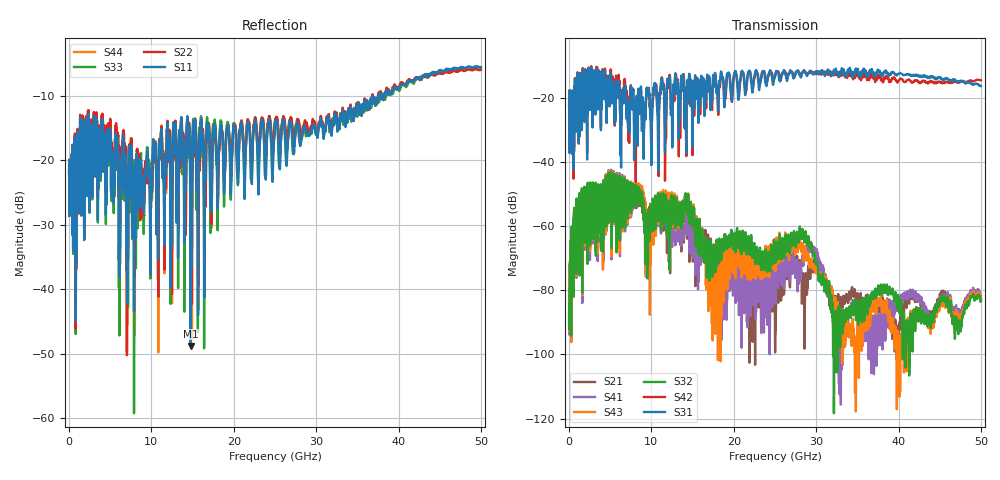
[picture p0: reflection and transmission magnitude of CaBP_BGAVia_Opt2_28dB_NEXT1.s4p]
!* Samtec Inc. NovaRay Examax Flyover System  *
!*  REV DATE  = 08/08/18  *
!*  TYPE  = TOUCHSTONE  *
!*  PORTS  = 4 port  *
!*  UNITS  = GHz  *
!*  DATA RANGE = DC  to 50 GHz; 10 MHz Step  *
!*  PARAMETER  = S  *
!*  FORMAT  = Real-Imaginary  *
!*  REFERENCE  = 50 ohms  *
!*  SOURCE  = HFSS  *
!*  VALIDATED  = No  *
!*  MANUFACTURER = SAMTEC  *
!*  INTERCONNECT = NVAx to EBCx to EBCx to NVAx  *
!*  [Full Channel NVAx to EBCx to EBCx to NVAx  with PCB Trace and BGA Via]  *
!*  BOUNDARY A  = Silicon BGA Ball Pad  *
!*  BOUNDARY B  = Silicon BGA Ball Pad  *
!*  NVAx (end a) ->>- (end b) NVAx  *
!*  Port 01 ->>- Port 02  *
!*  Port 03 ->>- Port 04  *
!***************************** CHANNEL MODEL ******************************************
# GHz S RI R 50
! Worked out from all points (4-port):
!   5000 points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, 10 MHz to 50 GHz, reference 50 ohm
!   strongest paths, dB at 10 MHz, 12.51 GHz, 25.01 GHz, 37.51 GHz, 50 GHz:
!     S31: -23.1, -28.5, -13.0, -11.3, -16.4
!     S42: -23.1, -22.9, -13.4, -12.9, -14.5
!     S32: -87.8, -59.5, -69.8, -78.9, -83.4
!     S43: -88.9, -57.6, -71.3, -83.6, -82.5
!     S41: -90.3, -63.2, -82.9, -89.0, -81.8
!     S21: -88.4, -62.3, -96.7, -84.9, -82.9
!   lowest |S11| = -48.8 dB at 14.75 GHz (marker M1), VSWR 1.01, Z = 49.7 - j0.221 ohm
!   |S11| at or under -10 dB: start of sweep to 37.51 GHz; 37.83997 GHz to 38.00552 GHz (165.6 MHz wide, 0.437 % of centre); 38.04261 GHz to 38.22467 GHz (182.1 MHz wide, 0.477 % of centre)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
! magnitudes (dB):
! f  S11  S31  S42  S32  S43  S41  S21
! 10 MHz  -22.1  -23.1  -23.1  -87.8  -88.9  -90.3  -88.4
! 1.02 GHz  -16.4  -13.2  -12.8  -53.7  -54.6  -55.6  -54.1
! 4.79 GHz  -20.3  -17.0  -15.2  -43.4  -42.9  -42.6  -42.8
! 14.75 GHz  -48.8  -22.0  -19.6  -54.8  -55.0  -62.5  -61.7
! 17.5 GHz  -15.4  -12.9  -14.0  -67.1  -74.6  -71.9  -67.8
! 27.09 GHz  -16.1  -12.2  -11.9  -64.8  -66.1  -72.1  -73.4
! 50 GHz  -5.6  -16.4  -14.5  -83.4  -82.5  -81.8  -82.9
